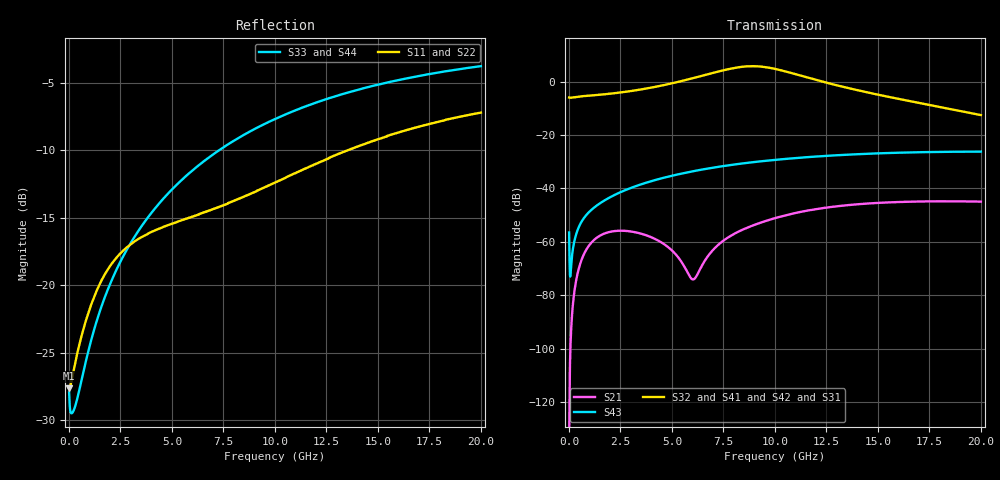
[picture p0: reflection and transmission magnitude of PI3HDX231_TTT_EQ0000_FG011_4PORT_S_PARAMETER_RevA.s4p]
! NPort=4 DATA=2000 NOISE=0 GROUPDELAY=0 COMPLEX_DATAFORMAT=POLAR
! NumOfBlock=1 NumOfParam=0
! .MODEL Smodel S TSTONEFILE=PI3HDX231_TTT_EQ0000_FG011_4PORT_S_PARAMETER_RevA.s4p TYPE=S
!  -- The above .MODEL line can be used for the S element in the netlist.
! The s parameter is extracted from the linear redriver, it is not bi-directional; only s(4,1)s(4,2) and s(3,1)s(3,2)
! should be the insertion loss
!Port definition:
!Port1 = input+
!Port2 = input-
!Port3 = output+
!Port4 = output-
# Hz S MA R  50
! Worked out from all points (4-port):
!   2000 points, 10 MHz to 20 GHz, reference 50 ohm
!   strongest paths, dB at 10 MHz, 5.01 GHz, 10.01 GHz, 15.01 GHz, 20 GHz:
!     S32: -5.9, -0.6, 4.8, -4.9, -12.5
!     S41: -5.9, -0.6, 4.7, -5.0, -12.6
!     S42: -5.9, -0.5, 4.7, -4.9, -12.3
!     S31: -5.9, -0.6, 4.5, -5.3, -12.7
!     S43: -56.5, -35.2, -29.3, -26.9, -26.2
!     S21: -134.8, -63.3, -51.1, -45.4, -44.9
!   lowest |S11| = -27.6 dB at 10 MHz (marker M1), VSWR 1.09, Z = 46 - j0.0776 ohm
!   |S11| at or under -10 dB: start of sweep to 13.55 GHz
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1e7  0.04152 -178.8  1.825e-07 -13.9  0 0.0  0 0.0
     1.825e-07 -14.0  0.04152 -178.8  0 0.0  0 0.0
     0.5041 -0.7  0.5041 179.3  0.04012 -3.2  0.0015 -70.3
     0.5041 179.3  0.5041 -0.7  0.0015 -70.3  0.04012 -3.2
2.19e9  0.1233 -139.7  0.001587 38.8  3.093e-12 -72.4  2.712e-12 -63.2
        0.001588 38.8  0.1233 -139.7  2.672e-12 -64.0  3.147e-12 -71.5
        0.5962 -16.7  0.606 163.5  0.1092 -90.9  0.00747 73.4
        0.6068 163.5  0.595 -15.9  0.007469 73.3  0.1092 -90.9
5.96e9  0.1791 -138.3  0.0001969 31.5  1.596e-09 164.7  6.166e-10 -163.0
        0.0002026 31.3  0.1789 -138.5  5.927e-10 -162.3  1.672e-09 164.4
        1.141 -66.6  1.144 112.5  0.2645 -105.3  0.02083 56.2
        1.141 112.1  1.159 -65.1  0.02076 56.1  0.2646 -105.3
7.94e9  0.2043 -133.6  0.001361 99.7  1.018e-08 101.4  3.756e-09 -179.8
        0.001356 99.1  0.2037 -133.8  3.669e-09 -177.9  1.071e-08 99.9
        1.761 -118.5  1.777 60.8  0.34 -110.5  0.02788 43.9
        1.765 60.4  1.799 -117.2  0.02777 43.9  0.3401 -110.6
9.37e9  0.228 -130.6  0.002346 87.8  2.472e-08 51.0  1.529e-08 138.1
        0.002331 87.3  0.2269 -130.8  1.506e-08 139.9  2.587e-08 48.4
        1.868 -171.8  1.905 7.4  0.3907 -114.1  0.0325 34.5
        1.888 7.0  1.91 -170.5  0.03237 34.6  0.3909 -114.2
1.152e10  0.2715 -128.3  0.003843 66.9  5.53e-08 -4.8  4.826e-08 61.2
          0.003813 66.4  0.2698 -128.4  4.787e-08 62.9  5.642e-08 -8.2
          1.169 122.6  1.212 -59.1  0.4594 -119.2  0.03854 20.6
          1.197 -59.4  1.197 124.2  0.03841 20.8  0.4594 -119.2
2e10  0.4354 -135.6  0.005717 -5.1  3.815e-07 -160.5  2.792e-07 -128.2
      0.005666 -5.2  0.4337 -135.4  2.8e-07 -127.3  3.733e-07 -163.1
      0.2315 -19.7  0.2364 152.9  0.6464 -135.0  0.04883 -32.3
      0.2334 153.6  0.2434 -18.1  0.04893 -32.0  0.6461 -135.0
